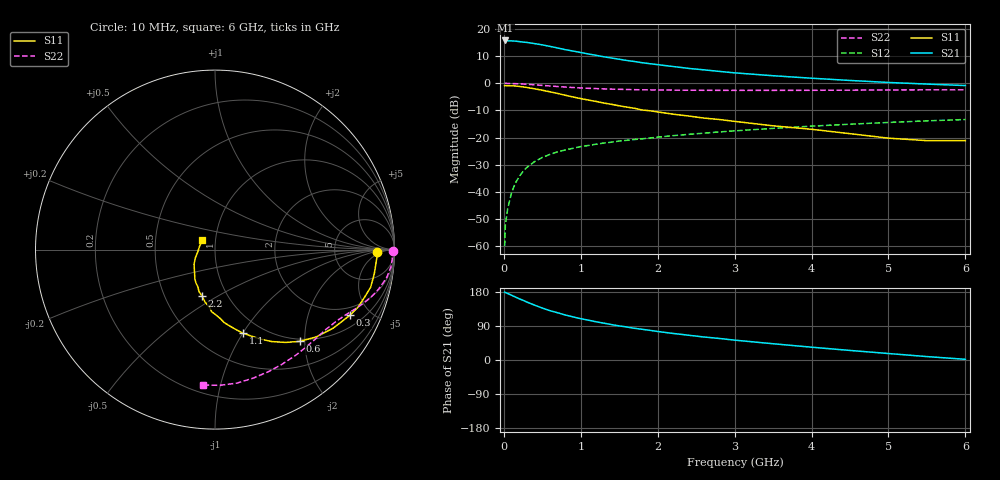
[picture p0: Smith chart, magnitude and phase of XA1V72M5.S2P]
! SIEMENS Discrete & RF Semiconductors
! BFY180
! Si NPN RF Bipolar Junction Transistor in MICRO-X
! VCE = 1.75 V  IC = 2.5 mA
! Common Emitter S-Parameters:  May  1997
# GHz  S  MA  R  50
!  f  S11  S21  S12  S22
! GHz  MAG  ANG  MAG  ANG  MAG  ANG  MAG  ANG
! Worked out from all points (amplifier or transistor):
!   36 points, 10 MHz to 6 GHz, reference 50 ohm
!   highest |S21| = 15.8 dB at 20 MHz (marker M1)
!   |S21| within 3 dB of that: start of sweep to 737.2 MHz
!   unconditionally stable (mu >= 1): 1.847 GHz to end of sweep
!   at 250 MHz: K = 0.17, MSG = 23.8 dB, |S12| = -32.4 dB
!   at 1.4 GHz: K = 0.86, MSG = 15.5 dB, |S12| = -21.7 dB
!   at 6 GHz: K = 1.12, MAG = 4.1 dB, |S12| = -13.3 dB
!   S11 on the Smith chart (normalised r, x): 10 MHz: 19, -3; 300 MHz: 1.54, -3.75; 600 MHz: 0.95, -1.89; 1.1 GHz: 0.82, -1.00; 2.2 GHz: 0.76, -0.43; 6 GHz: 0.86, +0.09
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0.01  0.9026 -0.8  6.03 179.2  0.001 79.2  0.9909 -0.3
0.02  0.9052 -1.7  6.147 178.0  0.0025 91.0  0.9999 -0.7
0.05  0.9005 -4.4  6.035 175.5  0.0049 84.1  0.991 -1.9
0.1  0.8976 -8.7  6.039 170.9  0.0096 85.2  0.9877 -3.8
0.2  0.8752 -17.5  5.865 161.6  0.0191 79.7  0.9768 -7.4
0.3  0.8364 -25.9  5.651 152.9  0.0283 74.1  0.9584 -10.7
0.4  0.791 -33.6  5.378 144.7  0.0361 70.3  0.937 -13.7
0.5  0.7446 -40.8  5.096 137.1  0.043 66.3  0.914 -16.3
0.6  0.6958 -47.3  4.776 130.1  0.0491 63.3  0.8921 -18.6
0.8  0.6014 -58.4  4.161 118.6  0.0592 58.2  0.8527 -22.5
1  0.5228 -67.2  3.687 109.0  0.0683 54.8  0.8208 -25.8
1.1  0.4905 -71.6  3.46 105.0  0.0716 53.3  0.8083 -27.1
1.3  0.4327 -79.2  3.078 97.2  0.0793 51.0  0.7883 -30.0
1.5  0.3847 -85.7  2.773 90.0  0.0863 49.4  0.7742 -32.8
1.7  0.3462 -93.1  2.514 83.6  0.0921 48.1  0.7623 -35.4
2.2  0.2697 -105.3  2.036 70.1  0.1085 44.7  0.7484 -42.3
2.6  0.2287 -114.6  1.767 60.7  0.1206 42.2  0.7425 -47.7
3  0.1988 -124.3  1.556 52.4  0.1329 39.6  0.7406 -53.0
3.5  0.1646 -134.1  1.377 42.9  0.1477 36.4  0.7399 -59.7
4.5  0.118 -157.7  1.127 25.2  0.1764 29.0  0.7469 -73.4
5.5  0.0878 167.4  0.967 9.0  0.2032 21.0  0.7567 -87.9
6  0.088 143.7  0.908 1.8  0.2152 16.7  0.7576 -95.2
